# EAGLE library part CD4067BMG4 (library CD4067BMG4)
IC MUX/DEMUX 1X16 24SOIC Source: Datasheet
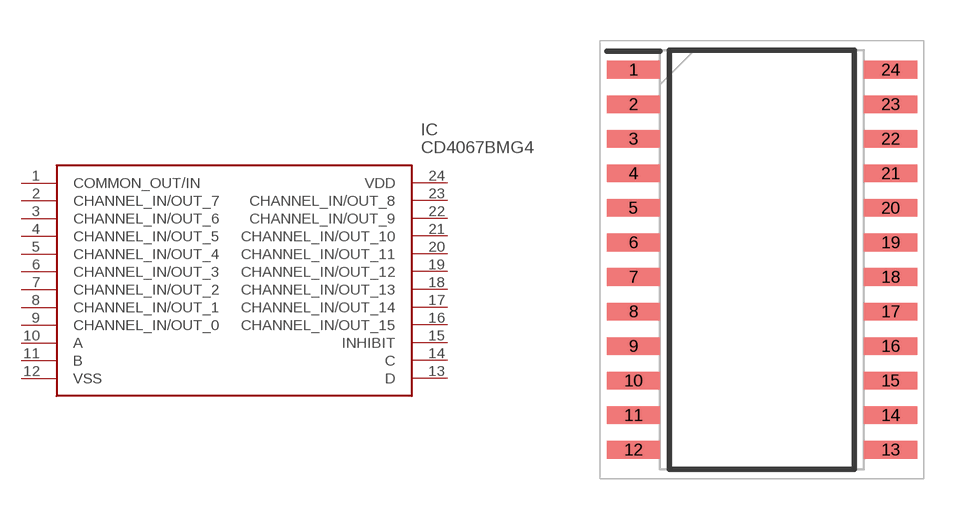
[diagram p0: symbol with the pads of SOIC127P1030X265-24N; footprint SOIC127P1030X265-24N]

Designator prefix IC

## CD4067BMG4 (Description: IC MUX/DEMUX 1X16 24SOIC; Height: 2.65mm; Manufacturer_Name: Texas Instruments; Manufacturer_Part_Number: CD4067BMG4)  [SOIC127P1030X265-24N]
1  COMMON_OUT/IN
2  CHANNEL_IN/OUT_7
3  CHANNEL_IN/OUT_6
4  CHANNEL_IN/OUT_5
5  CHANNEL_IN/OUT_4
6  CHANNEL_IN/OUT_3
7  CHANNEL_IN/OUT_2
8  CHANNEL_IN/OUT_1
9  CHANNEL_IN/OUT_0
10  A
11  B
12  VSS
13  D
14  C
15  INHIBIT
16  CHANNEL_IN/OUT_15
17  CHANNEL_IN/OUT_14
18  CHANNEL_IN/OUT_13
19  CHANNEL_IN/OUT_12
20  CHANNEL_IN/OUT_11
21  CHANNEL_IN/OUT_10
22  CHANNEL_IN/OUT_9
23  CHANNEL_IN/OUT_8
24  VDD

## Footprint SOIC127P1030X265-24N (pad centres in mm)
DW (R-PDSO-G24)
smd 1.95 x 0.65: 1 -4.725,6.985; 2 -4.725,5.715; 3 -4.725,4.445; 4 -4.725,3.175; 5 -4.725,1.905; 6 -4.725,0.635; 7 -4.725,-0.635; 8 -4.725,-1.905; 9 -4.725,-3.175; 10 -4.725,-4.445; 11 -4.725,-5.715; 12 -4.725,-6.985; 13 4.725,-6.985; 14 4.725,-5.715; 15 4.725,-4.445; 16 4.725,-3.175; 17 4.725,-1.905; 18 4.725,-0.635; 19 4.725,0.635; 20 4.725,1.905; 21 4.725,3.175; 22 4.725,4.445; 23 4.725,5.715; 24 4.725,6.985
